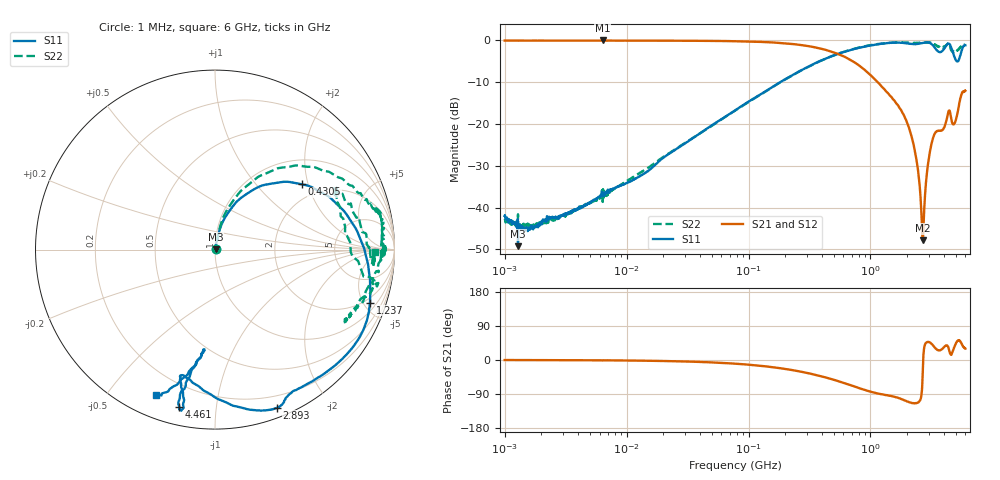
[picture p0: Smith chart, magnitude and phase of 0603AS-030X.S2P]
!s-Parameter Generated by FASTRON Sdn. Bhd.
!FASTRON P/N : 0603AS-030X
!Keysight Technologies: E5071C_MY46733604_B.14.02
!Date: Thu Nov 23 10:48:11 2023
!Version  :Rev01  Thu Nov 23 10:48:11 2023
!Data & Calibration Information:
!Freq  S11:SOLT2(ON)  S21:SOLT2(ON)  S12:SOLT2(ON)  S22:SOLT2(ON)
!PortZ  Port1:50+j0  Port2:50+j0
!When reading reference impedance value at option line is always used.
! Remarks : This data is being provided solely for informational purposes.
# Hz S dB R 50
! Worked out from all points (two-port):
!   1601 points, 1 MHz to 6 GHz, reference 50 ohm
!   highest |S21| = -0.02 dB at 6.378 MHz (marker M1); lowest = -47.9 dB at 2.687 GHz (marker M2)
!   |S21| within 3 dB of the highest: start of sweep to 516.8 MHz
!   lowest |S11| = -49.2 dB at 1.288 MHz (marker M3), VSWR 1.01, Z = 50.3 + j0.165 ohm
!   |S11| at or under -10 dB: start of sweep to 181.6 MHz
!   |S22| runs from -45.4 to -0.4 dB; largest |S21 - S12| = 0.0097
!   S11 on the Smith chart (normalised r, x): 1 MHz: 1.01, +0.01; 430.5 MHz: 1.59, +1.83; 1.237 GHz: 1.58, -5.58; 2.893 GHz: 0.09, -1.46; 4.461 GHz: 0.09, -0.79; 6 GHz: 0.10, -0.67
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1000000  -42.01 22.8  -0.05 -0.1  -0.06 -0.1  -42.69 24.1
1287650  -49.24 28.3  -0.06 -0.1  -0.05 -0.1  -41.61 14.8
4277066  -40.00 60.4  -0.06 -0.6  -0.06 -0.6  -40.02 60.4
6378092  -36.90 71.1  -0.02 -0.9  -0.08 -0.9  -38.66 71.6
1.823719e7  -29.08 77.9  -0.07 -2.4  -0.08 -2.4  -28.72 76.4
7.757876e7  -16.75 75.3  -0.19 -9.7  -0.20 -9.7  -16.81 77.1
3.307917e8  -5.87 47.1  -1.52 -37.0  -1.52 -37.0  -5.91 56.6
4.304579e8  -4.36 36.9  -2.28 -46.2  -2.28 -46.2  -4.38 49.4
7.811835e8  -1.87 5.4  -5.73 -72.5  -5.73 -72.6  -1.79 28.9
1.237427e9  -0.80 -18.9  -11.08 -90.4  -11.10 -90.5  -0.74 14.6
1.414819e9  -0.60 -24.7  -12.92 -94.2  -12.94 -94.2  -0.60 12.5
2.151902e9  -0.84 -55.8  -22.56 -112.7  -22.56 -112.6  -0.64 2.9
2.409089e9  -0.86 -62.7  -29.50 -113.1  -29.50 -113.0  -0.56 -0.7
2.599543e9  -0.70 -64.9  -39.80 -98.4  -39.83 -98.2  -0.52 -1.1
2.687444e9  -0.61 -65.6  -47.85 -22.0  -47.92 -21.9  -0.51 -1.3
2.760696e9  -0.54 -66.5  -40.10 33.7  -40.08 33.8  -0.57 -1.1
2.892548e9  -0.48 -68.6  -32.18 47.0  -32.16 47.0  -0.44 0.3
3.219478e9  -1.08 -82.1  -23.78 40.3  -23.76 40.2  -0.78 -4.9
3.786456e9  -2.77 -105.3  -21.57 26.9  -21.57 26.8  -1.67 -27.8
4.461108e9  -0.95 -102.8  -16.83 20.9  -16.86 20.7  -1.16 -10.1
5.048685e9  -4.88 -96.1  -18.60 46.0  -18.62 46.1  -2.55 27.3
6e9  -1.17 -112.1  -12.06 30.0  -12.06 30.1  -1.00 -1.0
